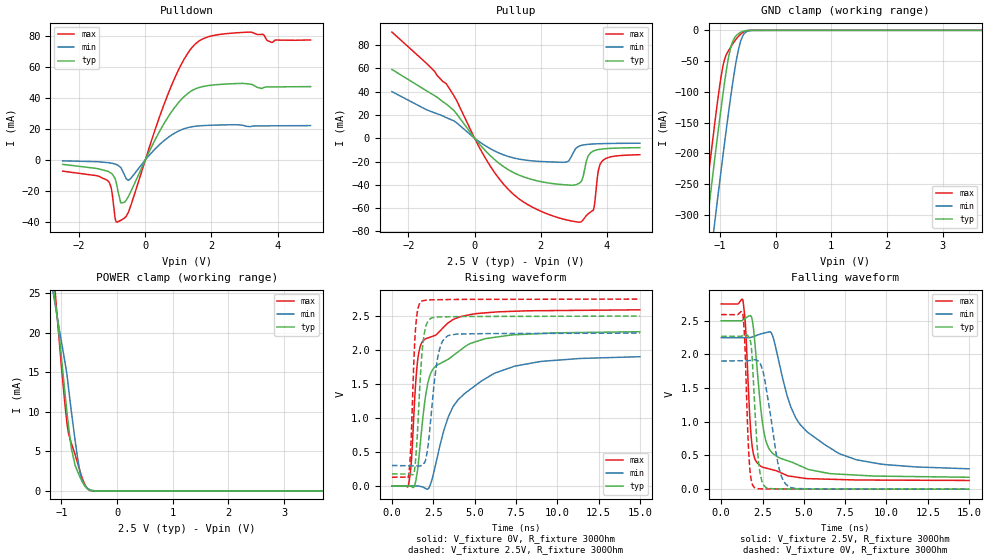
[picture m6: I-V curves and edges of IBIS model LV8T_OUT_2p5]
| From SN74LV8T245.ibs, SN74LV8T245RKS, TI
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[Model]   LV8T_OUT_2p5
Model_type   I/O
Polarity   Non-Inverting
Enable   Active-Low
Vinl = 0.65
Vinh = 1.28
Vmeas = 1.25
Vref = 0
Cref = 2pF
Rref = 100000
|   typ   min   max
C_comp   6.7pF   6.5pF   7pF
[Voltage Range]   2.5   2.25   2.75
[Temperature Range]   25   125   -40
[Pullup Reference]   2.5   2.25   2.75
[Pulldown Reference]   0   0   0
[Power Clamp Reference]   2.5   2.25   2.75
[GND Clamp Reference]   0   0   0
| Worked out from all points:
|   slope of the pulldown table from 0 to 0.375 V, typ, clamps not added: 23.2 ohm
|   slope of the pullup table from 0 to 0.375 V, typ, clamps not added: 31 ohm
|   GND clamp passes 1 mA (typ) near -0.56 V on its own axis
|   POWER clamp passes 1 mA (typ) near -0.61 V on its own axis
|   falling waveform, V_fixture 2.5V, R_fixture 300Ohm: 20-80 % time 730ps typ, 2.57ns min, 354ps max; typ from 2.5 V to 0.177 V
|   rising waveform, V_fixture 0V, R_fixture 300Ohm: 20-80 % time 1.38ns typ, 2.59ns min, 526ps max; typ from 0 V to 2.27 V
|   rising waveform, V_fixture 2.5V, R_fixture 300Ohm: 20-80 % time 340ps typ, 517ps min, 249ps max; typ from 0.177 V to 2.5 V
|   falling waveform, V_fixture 0V, R_fixture 300Ohm: 20-80 % time 337ps typ, 732ps min, 227ps max; typ from 2.27 V to 0 V
[Pulldown]
|   Voltage   I(typ)   I(min)   I(max)
-2.5V     -2.881mA   -614.4uA   -7.254mA
-1.145V   -7.279mA   -1.739mA   -13.2mA
-1.03V    -8.668mA   -2.108mA   -18.46mA
-904mV    -12.9mA    -2.768mA   -38.58mA
-736mV    -27.81mA   -5.139mA   -38.89mA
-505mV    -23.29mA   -13.1mA    -33.33mA
723.5mV   28.84mA    14.99mA    44.43mA
1.48V     45.41mA    21.55mA    74mA
2.046V    48.23mA    22.35mA    80.08mA
3.075V    49.02mA    21.56mA    82.24mA
3.832V    47mA       21.95mA    75.61mA
4.997V    47.22mA    22.09mA    77.21mA
[GND Clamp]
|   Voltage   I(typ)   I(min)   I(max)
-2.5V     -1.32A     -1.415A    -1.27A
-1.335V   -392.6mA   -495.4mA   -334.5mA
-1.23V    -311.6mA   -414.9mA   -253.3mA
-1.093V   -208.7mA   -311.7mA   -151.2mA
-1.009V   -147.7mA   -249.6mA   -93.35mA
-946mV    -104.1mA   -203.9mA   -58.53mA
-893.5mV  -70.5mA    -166.8mA   -41.26mA
-809.5mV  -29.07mA   -110mA     -27.75mA
-694mV    -7.468mA   -43.15mA   -12.67mA
-589mV    -1.77mA    -9.001mA   -3.449mA
-421mV    -17.94uA   -161.4uA   -14.88uA
8V        0A         0A         0A
[Pullup]
|   Voltage   I(typ)   I(min)   I(max)
-2.5V     59.08mA    40.04mA    91.16mA
-862mV    29.52mA    17.76mA    47mA
282.5mV   -9.367mA   -5.652mA   -14.98mA
870.5mV   -24.25mA   -14.19mA   -39.26mA
1.899V    -36.6mA    -19.75mA   -61.29mA
2.781V    -40.06mA   -20.41mA   -70.12mA
3.223V    -37.09mA   -6.189mA   -71.7mA
3.433V    -15.19mA   -5.22mA    -64.9mA
3.59V     -10.97mA   -4.898mA   -61.71mA
3.737V    -9.738mA   -4.714mA   -28.7mA
3.853V    -9.24mA    -4.613mA   -19.81mA
4.997V    -8.083mA   -4.249mA   -14.12mA
[POWER Clamp]
|   Voltage   I(typ)   I(min)   I(max)
-2.5V     105mA      84.61mA    129.9mA
-1.135V   25.15mA    24.47mA    27.24mA
-1.114V   24.01mA    23.6mA     25.38mA
-1.062V   21.19mA    21.42mA    20.77mA
-935.5mV  12.32mA    16.24mA    10.9mA
-883mV    8.871mA    13.65mA    7.695mA
-820mV    5.334mA    9.97mA     6.007mA
-757mV    3.316mA    6.557mA    4.656mA
-662.5mV  1.684mA    2.226mA    2.411mA
-589mV    715.9uA    794.8uA    961.3uA
-484mV    74.52uA    145.8uA    53.97uA
8V        0A         0A         0A
[Ramp]
R_load = 300
|   typ   min   max
dV/dt_r   1.36163/1.39462e-09   1.14105/2.5797e-09   1.55493/5.21191e-10
dV/dt_f   1.39373/7.24775e-10   1.1681/2.56478e-09   1.57228/3.53419e-10
[Falling Waveform]
V_fixture = 2.5V
V_fixture_min = 2.25V
V_fixture_max = 2.75V
R_fixture = 300Ohm
C_fixture = 0F
|   Time   V(typ)   V(min)   V(max)
0s        2.5V       2.249V     2.75V
1.31ns    2.511V     2.249V     2.808V
1.466ns   2.538V     2.249V     2.444V
1.848ns   2.542V     2.257V     692.3mV
2.33ns    1.359V     2.299V     353mV
2.63ns    793.4mV    2.319V     318.5mV
3.087ns   537.9mV    2.29V      289.3mV
4.498ns   377.2mV    1.066V     180.7mV
6.271ns   244.9mV    660.5mV    149.3mV
15ns      176.8mV    302.5mV    129.4mV
[Rising Waveform]
V_fixture = 0V
V_fixture_min = 0V
V_fixture_max = 0V
R_fixture = 300Ohm
C_fixture = 0F
|   Time   V(typ)   V(min)   V(max)
0s        72.1uV     207.2uV    29.98uV
1ns       1.494mV    143.1uV    7.855mV
1.18ns    -9.406mV   112uV      372.5mV
1.535ns   209.4mV    50.59uV    1.804V
1.966ns   1.2V       -27.52mV   2.155V
2.419ns   1.694V     90.83mV    2.199V
3.16ns    1.833V     833.7mV    2.343V
3.726ns   1.922V     1.176V     2.452V
6.072ns   2.182V     1.641V     2.555V
15ns      2.269V     1.902V     2.592V
[Rising Waveform]
V_fixture = 2.5V
V_fixture_min = 2.25V
V_fixture_max = 2.75V
R_fixture = 300Ohm
C_fixture = 0F
|   Time   V(typ)   V(min)   V(max)
0s        176.8mV    302.5mV    129.4mV
1.003ns   176.6mV    297.1mV    148.3mV
1.157ns   171.3mV    296.3mV    657.7mV
1.43ns    382mV      294.9mV    2.32V
1.777ns   1.82V      299.7mV    2.716V
1.96ns    2.249V     341.1mV    2.729V
2.181ns   2.426V     586.9mV    2.737V
2.768ns   2.486V     1.888V     2.74V
3.368ns   2.489V     2.207V     2.742V
15ns      2.5V       2.249V     2.75V
[Falling Waveform]
|Gnd
V_fixture = 0V
V_fixture_min = 0V
V_fixture_max = 0V
R_fixture = 300Ohm
C_fixture = 0F
|   Time   V(typ)   V(min)   V(max)
0s        2.269V     1.902V     2.592V
1.304ns   2.28V      1.906V     2.609V
1.424ns   2.293V     1.907V     2.21V
1.707ns   2.234V     1.909V     382.9mV
2.025ns   1.252V     1.921V     20.26mV
2.259ns   411.9mV    1.895V     6.019mV
2.515ns   84.17mV    1.763V     3.924mV
3.491ns   4.051mV    321.6mV    2.329mV
4.079ns   2.907mV    39.26mV    2.211mV
15ns      72.09uV    207.3uV    29.94uV
